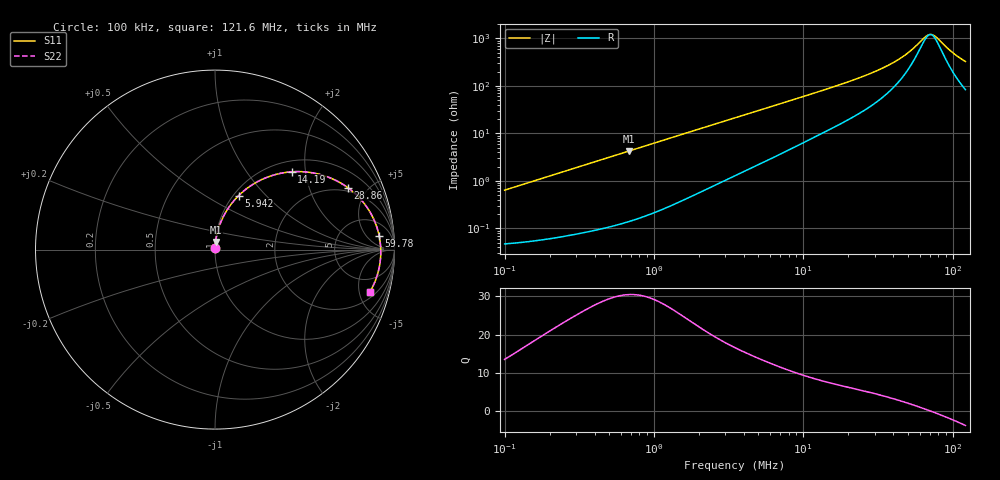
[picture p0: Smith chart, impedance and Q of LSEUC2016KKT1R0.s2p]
! LSEUC2016KKT1R0  S-PARAMETER MODEL  ( General Type )
! Model Generated by TAIYO YUDEN Corporation (http://www.ty-top.com)
! Version 1.0
! TAIYO YUDEN Control No. 211126
! Copyright(c) 2021 TAIYO YUDEN CO.,LTD. All Rights Reserved.
! Product Description (link to TY-COMPAS)
! https://ds.yuden.co.jp/TYCOMPAS/or/detail?pn=LSEUC2016KKT1R0M&u=M
! Products Name : Inductors
! Characteristics :
!  Inductance : 1.0 uH , SRF(min) : -Hz , DC Resistance(max) : 0.048 Ohm
!  Rated Current : Saturation :4100 mA , Temp Rise : 3500 mA (40 degC)
!  Case Size : 2.0 x 1.6 / 0.079 x 0.063 [mm/inch] , Thickness : 1 / 0.039 [mm/inch]
!  (Conditions: Temperature = 25 degC , DC Bias Current/Voltage = 0A / 0V)
! External Node Assignments :
!  1  o---GGG---o  2
! GND o---------o GND
! Frequency Range : 0.1MHz  -  121.638923MHz  [ 402 STEP ]
# MHz S RI R 50
! Freq[MHz].  S11 Real  S11 Imag  S21 Real  S21 Imag  S12 Real  S12 Imag  S22 Real  S22 Imag
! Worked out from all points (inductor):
!   401 points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, 100 kHz to 121.6 MHz, reference 50 ohm
!   read as one part in series: L = 1.01 uH near 103.6 kHz
!   highest Q = 30.5 at 680.7 kHz (marker M1), where L = 994 nH
!   self-resonance near 70.82 MHz
!   S11 on the Smith chart (normalised r, x): 100 kHz: 1.00, +0.01; 5.942 MHz: 1.06, +0.71; 14.19 MHz: 1.22, +1.68; 28.86 MHz: 1.78, +3.69; 59.78 MHz: 12, +12; 121.6 MHz: 2.66, -6.32
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0.1  0.000511 0.00636  0.9995 -0.00636  0.9995 -0.00636  0.000511 0.00636
0.328662  0.00122 0.0206  0.9988 -0.0206  0.9988 -0.0206  0.00122 0.0206
0.680722  0.00319 0.0423  0.9968 -0.0423  0.9968 -0.0423  0.00319 0.0423
1.080188  0.0068 0.0665  0.9932 -0.0665  0.9932 -0.0665  0.0068 0.0665
2.011144  0.0205 0.1207  0.9795 -0.1207  0.9795 -0.1207  0.0205 0.1207
3.550168  0.0559 0.2012  0.9441 -0.2012  0.9441 -0.2012  0.0559 0.2012
5.941782  0.132 0.3011  0.868 -0.3011  0.868 -0.3011  0.132 0.3011
8.179843  0.2147 0.3658  0.7853 -0.3658  0.7853 -0.3658  0.2147 0.3658
11.46267  0.3362 0.418  0.6638 -0.418  0.6638 -0.418  0.3362 0.418
14.18529  0.4274 0.4334  0.5726 -0.4334  0.5726 -0.4334  0.4274 0.4334
20.23447  0.5896 0.4173  0.4104 -0.4173  0.4104 -0.4173  0.5896 0.4173
28.86326  0.7397 0.3455  0.2603 -0.3455  0.2603 -0.3455  0.7397 0.3455
37.67347  0.8287 0.2604  0.1713 -0.2604  0.1713 -0.2604  0.8287 0.2604
48.30734  0.8867 0.1644  0.1133 -0.1644  0.1133 -0.1644  0.8867 0.1644
59.78129  0.9151 0.0744  0.0849 -0.0744  0.0849 -0.0744  0.9151 0.0744
67.69461  0.9225 0.02  0.0775 -0.02  0.0775 -0.02  0.9225 0.02
71.399  0.9236 -0.0036  0.0764 0.0036  0.0764 0.0036  0.9236 -0.0036
73.98054  0.9236 -0.0194  0.0764 0.0194  0.0764 0.0194  0.9236 -0.0194
78.02891  0.9226 -0.0431  0.0774 0.0431  0.0774 0.0431  0.9226 -0.0431
100.0537  0.9006 -0.1533  0.0994 0.1533  0.0994 0.1533  0.9006 -0.1533
113.2979  0.8785 -0.2071  0.1215 0.2071  0.1215 0.2071  0.8785 -0.2071
121.6389  0.8626 -0.237  0.1374 0.237  0.1374 0.237  0.8626 -0.237
